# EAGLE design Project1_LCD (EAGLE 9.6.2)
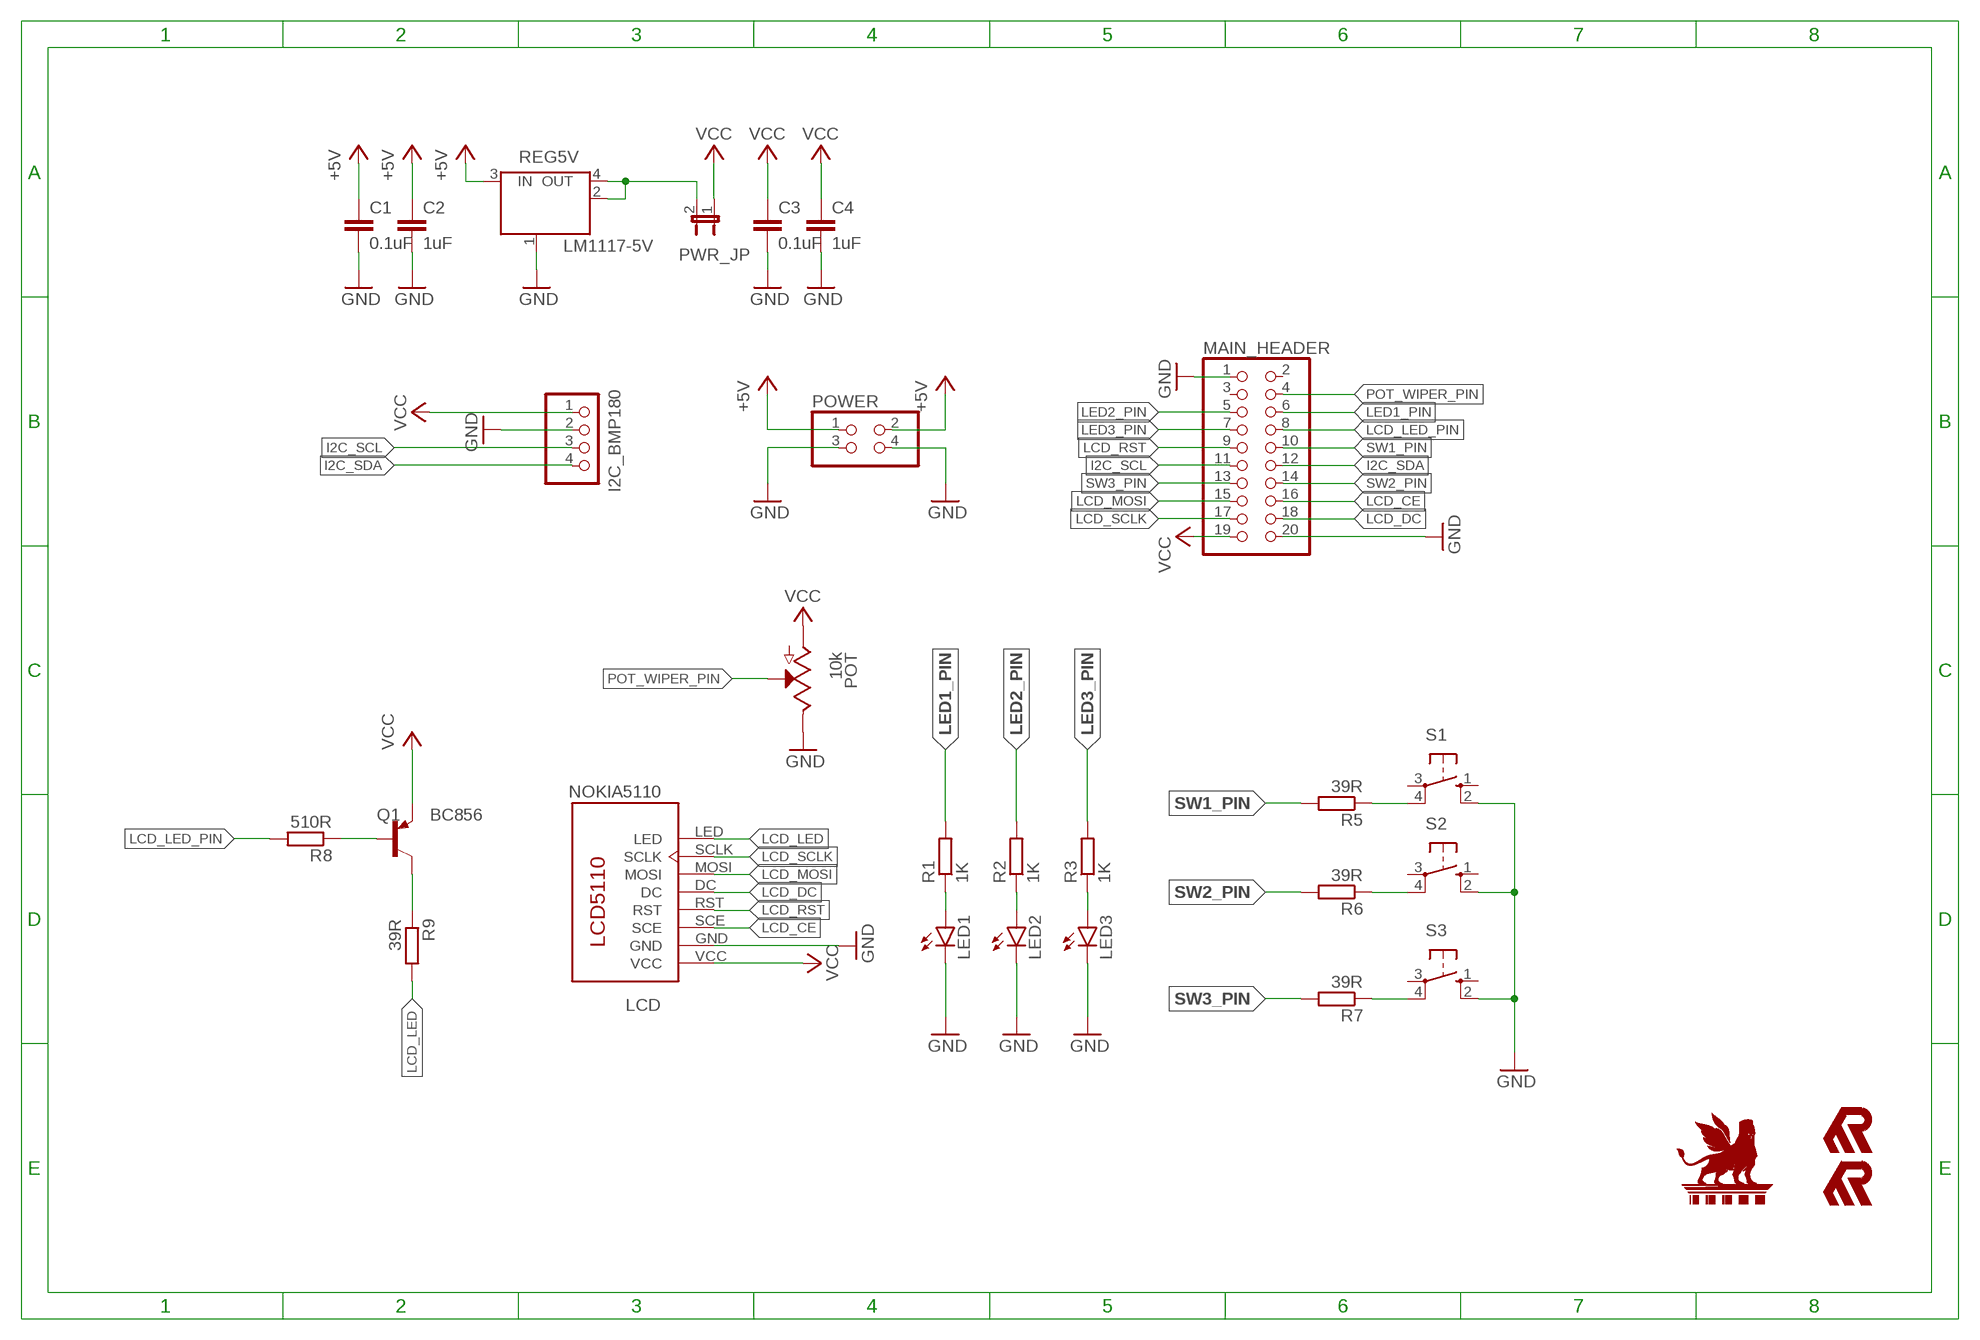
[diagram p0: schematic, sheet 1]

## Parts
C1  0.1uF  C-EUC0805  [C0805]
C2  1uF  C-EUC0805  [C0805]
C3  0.1uF  C-EUC0805  [C0805]
C4  1uF  C-EUC0805  [C0805]
I2C_BMP180  PINHD-1X4  [1X04]
LCD  NOKIA5110  [PCD8544]
LED1  LED5MM  [LED5MM]
LED2  LED5MM  [LED5MM]
LED3  LED5MM  [LED5MM]
MAIN_HEADER  PINHD-2X10  [2X10]
POT  10k  POTENTIOMETER-PTH-9MM-1/20W-20%-KIT  [POT-PTH-ALPS-KIT]
POWER  PINHD-2X2  [2X02]
PWR_JP  JP1E  [JP1]
Q1  BC856  BC856ASMD  [SOT23-BEC]
R1  1K  R-EU_0207/10  [0207/10]
R2  1K  R-EU_0207/10  [0207/10]
R3  1K  R-EU_0207/10  [0207/10]
R5  39R  R-EU_0207/10  [0207/10]
R6  39R  R-EU_0207/10  [0207/10]
R7  39R  R-EU_0207/10  [0207/10]
R8  510R  R-EU_0207/10  [0207/10]
R9  39R  R-EU_0207/10  [0207/10]
REG5V  LM1117-5V  MC33269ST-3.3T3  [SOT223]
S1  40-XX  [B3F-40XX]
S2  40-XX  [B3F-40XX]
S3  40-XX  [B3F-40XX]
U$1  LAMASSU_SMALL_SIZE24  [LAMASSU_SMALL_24MM]
U$2  MR_SMALL_SIZE12  [MR_SMALL_12MM]
U$3  MR_SMALL_SIZE7  [MR_SMALL_7MM]

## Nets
+5V [POWER]: C1.1 C2.1 POWER.1 POWER.2 REG5V.3(IN)
BQ1 [LCD]: Q1.B R8.1
GND [POWER]: C1.2 C2.2 C3.2 C4.2 I2C_BMP180.2 LCD.GND LED1.K(C) LED2.K(C) LED3.K(C) MAIN_HEADER.1 MAIN_HEADER.20 POT.P$1(E) POWER.3 POWER.4 REG5V.1(GND/ADJ) S1.2(S1) S2.2(S1) S3.2(S1)
I2C_SCL: I2C_BMP180.3 MAIN_HEADER.11
I2C_SDA: I2C_BMP180.4 MAIN_HEADER.12
LCD_CE [LCD]: LCD.SCE MAIN_HEADER.16
LCD_DC [LCD]: LCD.DC MAIN_HEADER.18
LCD_LED [LCD]: LCD.LED R9.2
LCD_LED_PIN [LCD]: MAIN_HEADER.8 R8.2
LCD_MOSI [LCD]: LCD.MOSI MAIN_HEADER.15
LCD_RST [LCD]: LCD.RST MAIN_HEADER.9
LCD_SCLK [LCD]: LCD.SCLK MAIN_HEADER.17
LED1_PIN: MAIN_HEADER.6 R1.2
LED2_PIN: MAIN_HEADER.5 R2.2
LED3_PIN: MAIN_HEADER.7 R3.2
N$3: LED3.A R3.1
N$4: LED2.A R2.1
N$5: LED1.A R1.1
N$6: R5.1 S1.4(P1)
N$7: R6.1 S2.4(P1)
N$8: R7.1 S3.4(P1)
POT_WIPER_PIN: MAIN_HEADER.4 POT.P$2(S)
REG_OUT [POWER]: PWR_JP.2 REG5V.2(OUT) REG5V.4(OUT)
RQ1 [LCD]: Q1.C R9.1
SW1_PIN: MAIN_HEADER.10 R5.2
SW2_PIN: MAIN_HEADER.14 R6.2
SW3_PIN: MAIN_HEADER.13 R7.2
VCC [POWER]: C3.1 C4.1 I2C_BMP180.1 LCD.VCC MAIN_HEADER.19 POT.P$3(A) PWR_JP.1 Q1.E
Unconnected: LCD.P$9(NC) LCD.P$10(NC) LCD.P$11(NC) LCD.P$12(NC) LCD.P$13(NC) LCD.P$14(NC) LCD.P$15(NC) LCD.P$16(NC) MAIN_HEADER.2 MAIN_HEADER.3 S1.1(S) S1.3(P) S2.1(S) S2.3(P) S3.1(S) S3.3(P)

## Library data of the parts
C1-C4 = rcl:C-EU: CAPACITOR, European symbol; SPICEPREFIX: C
I2C_BMP180 = pinhead:PINHD-1X4: PIN HEADER
LCD = Rawashdeh_Eagle_Display:NOKIA5110: LCD Nokia 5110 Nokia5110 ased on PCD8544 display driver
LED1-LED3 = led:LED: LED
MAIN_HEADER = pinhead:PINHD-2X10: PIN HEADER
POT = SparkFun-Resistors:POTENTIOMETER: Potentiometer (Pot) Three-terminal potentiometers, with an adjustable wiper and two adjustable resistors. A pot can be used to create a configurable voltage divider, or as a variable resistor. Variants ALPS_POT and ALPS_POT_KIT - PTH, breadboard compatible, 9mm square pots Rotary Potentiometer -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; PROD_ID: RES-09177; SF_SKU: COM-09288
POWER = pinhead:PINHD-2X2: PIN HEADER
PWR_JP = jumper:JP1E: JUMPER
Q1 = transistor-pnp:BC856*: PNP Transistror
R1-R3 R5-R9 = rcl:R-EU_: RESISTOR, European symbol; SPICEPREFIX: R
REG5V = linear:MC33269ST*: Adjustable Output Low Dropout Voltage Regulator 800 mA Source: http://www.onsemi.com/pub/Collateral/MC33269-D.PDF
S1-S3 = switch-omron:40-XX: OMRON SWITCH; MF: OMRON COMPONENTS USA; MPN: B3F-4000; OC_FARNELL: 176434; OC_NEWARK: 36K3105
U$1 = Rawashdeh_Eagle_Logo:LAMASSU_SMALL_SIZE: lamassu Rawashdeh Logo small sizes
U$2 U$3 = Rawashdeh_Eagle_Logo:MR_SMALL_SIZE: MR Mohannad Rawashdeh Logo 7,12 mm

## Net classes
0 default: width 0.254 mm, drill 0.406 mm, clearance 0.305 mm
1 POWER: width 0.406 mm, drill 0.406 mm, clearance 0.305 mm
2 LCD: width 0.254 mm, drill 0.406 mm, clearance 0.305 mm

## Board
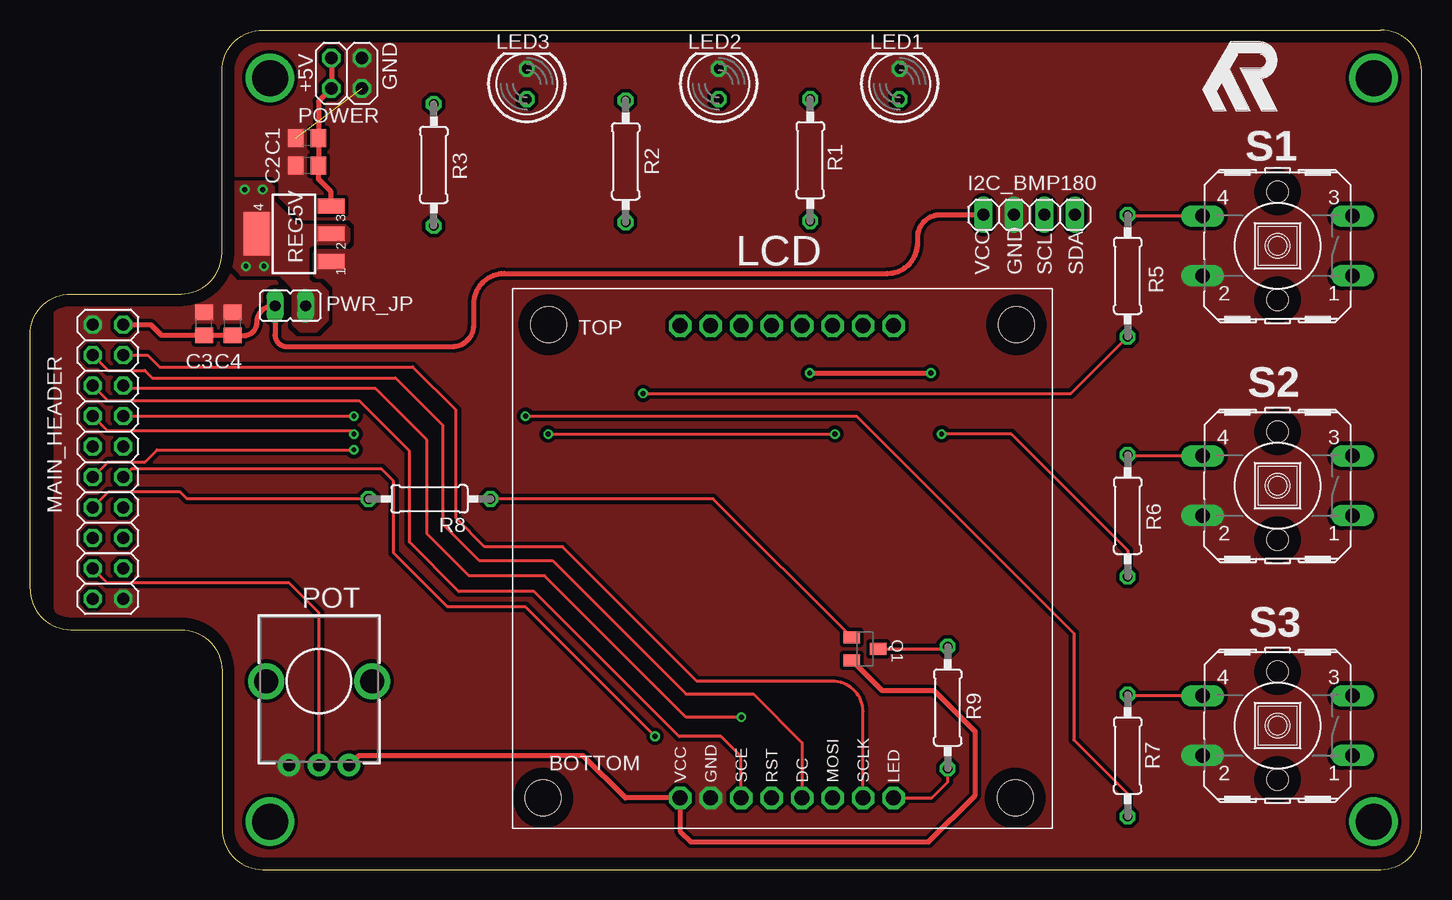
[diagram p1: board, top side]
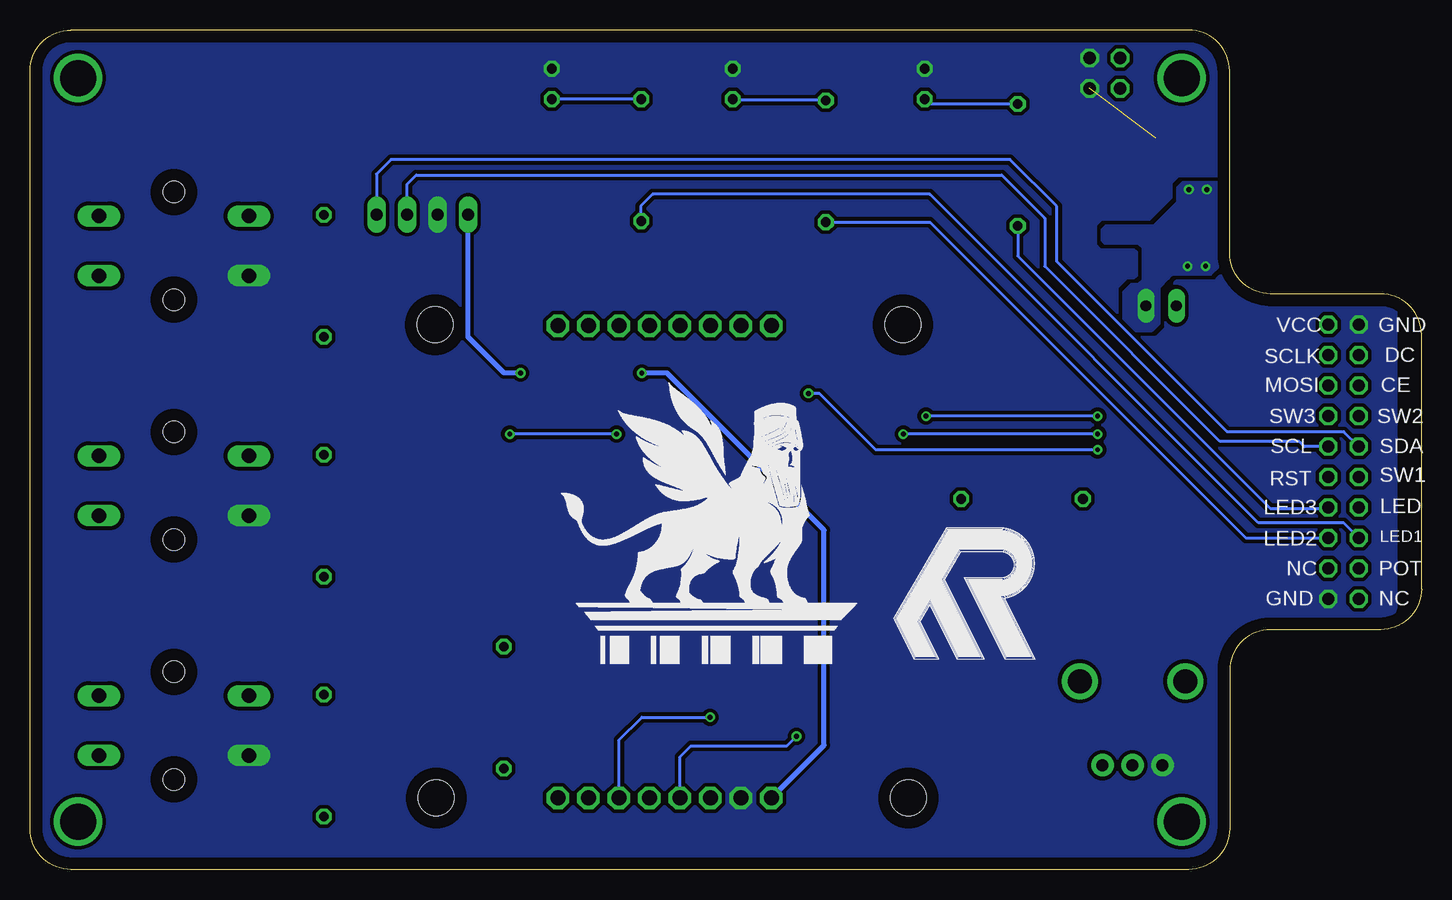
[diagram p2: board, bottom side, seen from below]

Size 116 x 70 mm. Coordinates in mm from the lower left corner, seen from the top.
Outline: 0,23.41 0,44.59 arc-90 3.41,48 12.59,48 arc90 16,51.41 16,66.59 arc-90 19.41,70 112.59,70 arc-90 116,66.59 116,3.41 arc-90 112.59,0 19.41,0 arc-90 16,3.41 16,16.59 arc90 12.59,20 3.41,20 arc-90 0,23.41
Copper layers (1*16): Top 0.035mm / dielectric 1.5mm / Bottom 0.035mm
Design rules "default": minimum track width 6mil, minimum drill 0.35mm, track to track 6mil, track to pad 6mil, pad to pad 6mil, via to via 6mil, smd to smd 6mil, copper to edge 40mil, drill to drill 6mil, minimum pad ring 10mil, minimum via ring 8mil, stop-mask expansion 4mil, vias tented up to drill 0mil, thermal gap 10mil

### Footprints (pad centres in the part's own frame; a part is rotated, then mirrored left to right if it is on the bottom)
C0805 = smd 1.3 x 1.5: 1 -0.95,0; 2 0.95,0
1X04 = drill 1.016 long: 1 -3.81,0; 2 -1.27,0; 3 1.27,0; 4 3.81,0
PCD8544 = drill 1.25 octagon: DC 24.13,2.54; GND 16.51,2.54; LED 31.75,2.54; MOSI 26.67,2.54; P$9 13.97,41.91; P$10 16.51,41.91; P$11 19.05,41.91; P$12 21.59,41.91; P$13 24.13,41.91; P$14 26.67,41.91; P$15 29.21,41.91; P$16 31.75,41.91; RST 21.59,2.54; SCE 19.05,2.54; SCLK 29.21,2.54; VCC 13.97,2.54 | hole 3: 2.54,2.54; 41.91,2.54; 3,42; 42,42
LED5MM = drill 0.813 octagon: A -1.27,0; K 1.27,0
2X10 = drill 1.016 octagon: 1 -11.43,-1.27; 2 -11.43,1.27; 3 -8.89,-1.27; 4 -8.89,1.27; 5 -6.35,-1.27; 6 -6.35,1.27; 7 -3.81,-1.27; 8 -3.81,1.27; 9 -1.27,-1.27; 10 -1.27,1.27; 11 1.27,-1.27; 12 1.27,1.27; 13 3.81,-1.27; 14 3.81,1.27; 15 6.35,-1.27; 16 6.35,1.27; 17 8.89,-1.27; 18 8.89,1.27; 19 11.43,-1.27; 20 11.43,1.27
POT-PTH-ALPS-KIT = drill 1 pad 1.88: P$1 7,-2.5; P$2 7,0; P$3 7,2.5 | drill 2: P$4 0,-4.4; P$5 0,4.4
2X02 = drill 1.016 octagon: 1 -1.27,-1.27; 2 -1.27,1.27; 3 1.27,-1.27; 4 1.27,1.27
JP1 = drill 0.914 long: 1 0,-1.27; 2 0,1.27
SOT23-BEC = smd 1 x 1.4: B -0.95,-1.1; C 0,1.1; E 0.95,-1.1
0207/10 = drill 0.813 octagon: 1 -5.08,0; 2 5.08,0
SOT223 = smd 1.219 x 2.235: 1 -2.311,-3.099; 2 0,-3.099; 3 2.311,-3.099 | smd 3.6 x 2.2: 4 0,3.099
B3F-40XX = drill 1.194 long: 1 -6.248,2.489; 2 6.248,2.489; 3 -6.248,-2.489; 4 6.248,-2.489 | hole 1.803: 0,-4.496; 0,4.496

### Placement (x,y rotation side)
C1  23.1,61 180 top
C2  23.1,58.7 180 top
C3  14.5,45.5 90 top
C4  16.9,45.5 90 top
I2C_BMP180  83.3,54.6 0 top
LCD  40.23,3.43 0 top
LED1  72.5,65.5 90 top
LED2  57.42,65.5 90 top
LED3  41.42,65.5 90 top
MAIN_HEADER  6.5,34 90 top
POT  24.1,15.7 270 top
POWER  26.4,66.4 0 top
PWR_JP  21.7,47 270 top
Q1  69.6,18.4 270 top
R1  65.04,59.15 270 top
R2  49.66,59.05 270 top
R3  33.66,58.75 270 top
R5  91.5,49.5 270 top
R6  91.5,29.5 270 top
R7  91.5,9.5 270 top
R8  33.3,30.9 180 top
R9  76.5,13.5 270 top
REG5V  22,53 90 top
S1  104,52 180 top
S2  104,32 180 top
S3  104,12 180 top
U$1  58.7,23.9 0 bottom
U$2  37,20.9 0 bottom
U$3  101.1,65.9 0 top

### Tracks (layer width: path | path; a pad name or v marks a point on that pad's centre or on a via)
+5V
  Top 0.406: POWER.2 POWER.1 24.05,64.05 C1.1 C2.1 24.05,57.55 25.1,56.5 REG5V.3
BQ1
  Top 0.254: Q1.B 56.95,30.9 R8.1
GND  (1 unrouted)
  pour Top (isolate 0.305, rank 2, no thermals): 3.3,47.7 12.5,47.7 arc90 16.4,51.6 16.4,66.8 arc-90 19.5,69.9 111.9,69.9 arc-90 115.5,66.3 115.5,3.9 arc-90 112,0.4 20.2,0.4 arc-90 16.5,4.1 16.5,16.3 arc90 12.1,20.7 3.5,20.7 arc-90 2.1,22.1 2.1,46.5 arc-90
  pour Bottom (isolate 0.254, rank 2, no thermals): 3.3,47.7 12.5,47.7 arc90 16.4,51.6 16.4,66.8 arc-90 19.5,69.9 111.9,69.9 arc-90 115.5,66.3 115.5,3.9 arc-90 112,0.4 20.2,0.4 arc-90 16.5,4.1 16.5,16.3 arc90 12.1,20.7 3.5,20.7 arc-90 2.1,22.1 2.1,46.5 arc-90
I2C_SCL
  Bottom 0.254: MAIN_HEADER.11 9.77,35.27 10.2,35.7 16.8,35.7 31.4,50.3 31.4,54.3 35,57.9 83.8,57.9 84.57,57.13 I2C_BMP180.3
I2C_SDA
  Bottom 0.254: MAIN_HEADER.12 6.46,36.5 16.2,36.5 30.4,50.7 30.4,55.3 34.3,59.2 85.9,59.2 87.11,57.99 I2C_BMP180.4
LCD_CE
  Top 0.254: MAIN_HEADER.16 6.48,39.1 27.42,39.1 31.63,34.9 31.63,27.3 35.74,23.18 42.04,23.18 54.12,11.1 57.6,11.1 59.28,9.42 LCD.SCE
LCD_DC
  Top 0.254: MAIN_HEADER.18 6.52,41.6 9.56,41.6 10.17,41 30.47,41 34.41,37.06 34.41,28.8 37.45,25.76 43.55,25.76 54.67,14.63 60.31,14.63 64.36,10.58 LCD.DC
LCD_LED
  Top 0.254: LCD.LED 75.17,5.97 76.5,7.3 R9.2
LCD_LED_PIN
  Top 0.254: R8.2 13.1,30.9 12.5,31.5 6.54,31.5 MAIN_HEADER.8
LCD_MOSI  (via drill 0.41)
  Top 0.254: v59.3,12.7 54.7,12.7 42.9,24.5 36.6,24.5 33.1,28 33.1,35.8 28.8,40.1 8.02,40.1 MAIN_HEADER.15
  Bottom 0.254: LCD.MOSI 66.9,10.8 65,12.7 v59.3,12.7
LCD_RST  (via drill 0.41)
  Top 0.254: v52.1,11.1 41.3,21.9 34.8,21.9 30.3,26.4 30.3,32.4 29.3,33.4 8.44,33.4 MAIN_HEADER.9
  Bottom 0.254: LCD.RST 61.82,9.38 60.9,10.3 52.9,10.3 v52.1,11.1
LCD_SCLK
  Top 0.254: LCD.SCLK 69.44,13.16 arc90 66.9,15.7 55.6,15.7 44.4,26.9 37.9,26.9 35.5,29.3 35.5,38.3 31.9,41.9 10.8,41.9 9.81,42.89 MAIN_HEADER.17
LED1_PIN
  Bottom 0.254: MAIN_HEADER.6 6.48,28.9 13.6,28.9 41,56.3 64.1,56.3 65.1,55.3 65.1,54.13 R1.2
LED2_PIN
  Bottom 0.254: R2.2 40.97,53.97 14.65,27.65 MAIN_HEADER.5
LED3_PIN
  Bottom 0.254: R3.2 33.66,51.16 12.6,30.1 7.86,30.1 MAIN_HEADER.7
N$3
  Bottom 0.254: R3.1 41.02,63.83 LED3.A
N$4
  Bottom 0.254: R2.1 57.32,64.13 LED2.A
N$5
  Bottom 0.254: R1.1 LED1.A
N$6
  Top 0.254: S1.4 91.59,54.49 R5.1
N$7
  Top 0.254: S2.4 91.59,34.49 R6.1
N$8
  Top 0.254: S3.4 91.59,14.49 R7.1
N$9  (via drill 3)
  other vias: 112,4
N$10  (via drill 3)
  other vias: 112,66
N$11  (via drill 3)
  other vias: 20,66
N$12  (via drill 3)
  other vias: 20,4
POT_WIPER_PIN
  Top 0.254: POT.P$2 24.1,21.4 21.6,23.9 6.44,23.9 MAIN_HEADER.4
REG_OUT  (via drill 0.41)
  other vias: 18,50.3 19.5,50.3 19.4,56.7 17.9,56.7
  pour Top (isolate 0.406, no thermals): 26.1,53.7 23.6,53.7 22.3,53.7 20.9,55.1 20.3,55.7 20.3,56.1 20.3,56.9 20.1,57.1 19.9,57.3 16.7,57.3 16.6,57.3 16.3,57 16.3,50.9 17,50.2 17.6,49.6 19.5,49.6 20.8,49.6 21.1,49.3 21.9,48.5 21.9,47.8 21.9,45.5 22.5,44.9 23.4,44.9 23.9,44.9 24.8,45.8 24.8,48.2 24.2,48.8 23.6,48.8 23.2,49.2 23.2,50.8 23.2,51.8 23.6,52.2 26.4,52.2 26.5,52.3 26.6,52.4 26.6,53.4 26.3,53.7
  pour Bottom (isolate 0.254, no thermals): 26.1,53.7 23.6,53.7 22.3,53.7 20.9,55.1 20.3,55.7 20.3,56.1 20.3,56.9 20.1,57.1 19.9,57.3 16.7,57.3 16.6,57.3 16.3,57 16.3,50.9 17,50.2 17.6,49.6 19.5,49.6 20.8,49.6 21.1,49.3 21.9,48.5 21.9,47.8 21.9,45.5 22.5,44.9 23.4,44.9 23.9,44.9 24.8,45.8 24.8,48.2 24.2,48.8 23.6,48.8 23.2,49.2 23.2,50.8 23.2,51.8 23.6,52.2 26.4,52.2 26.5,52.3 26.6,52.4 26.6,53.4 26.3,53.7
RQ1
  Top 0.254: Q1.C 76.32,18.4 R9.1
SW1_PIN  (via drill 0.41)
  Top 0.254: MAIN_HEADER.10 6.5,34 9.6,34 10.6,35 v27,35 | v51.1,39.7 86.78,39.7 R5.2
  Bottom 0.254: v27,35 45.5,35 50.2,39.7 v51.1,39.7
SW2_PIN  (via drill 0.41)
  Top 0.254: MAIN_HEADER.14 6.44,36.6 26.7,36.6 v27,36.3 | v76,36.3 81.8,36.3 91.5,26.6 R6.2 | v43.2,36.3 v67.1,36.3
  Bottom 0.254: v27,36.3 v43.2,36.3 | v67.1,36.3 v76,36.3
SW3_PIN  (via drill 0.41)
  Top 0.254: MAIN_HEADER.13 v26.99,37.81 v27,37.8 | v41.3,37.8 68.9,37.8 87,19.7 87,10.8 91.5,6.3 R7.2
  Bottom 0.254: v27,37.8 v41.3,37.8
VCC  (via drill 0.41)
  Top 0.406: MAIN_HEADER.19 10.07,45.43 10.95,44.55 C3.1 C4.1 arc90 16.95,44.5 17.8,44.5 arc90 18.9,45.6 arc-90 20.3,47 PWR_JP.1 20.43,44.57 arc90 21.4,43.6 35.2,43.6 arc90 37,45.4 37,47.16 arc-90 39.54,49.7 71.46,49.7 arc90 74,52.24 74,52.7 arc-90 75.9,54.6 I2C_BMP180.1 | POT.P$3 27.4,9.5 46.1,9.5 49.63,5.97 LCD.VCC 54.2,3.2 55.1,2.3 74.9,2.3 78.8,6.2 78.8,11.5 75.4,14.9 71.05,14.9 Q1.E | v65,41.4 v75.1,41.4
  Bottom 0.406: LCD.VCC 49.8,10.37 49.8,28.3 62.9,41.4 v65,41.4 | I2C_BMP180.1 79.5,44.4 76.5,41.4 v75.1,41.4

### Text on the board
tNames: +5V | GND | VCC | GND | SCL | SDA
bNames: GND | VCC | DC | SCLK | CE | MOSI | SW2 | SW3 | SDA | SCL | SW1 | RST | LED | LED3 | LED1 | LED2 | POT | NC | NC | GND

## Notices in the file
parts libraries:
SparkFun-Resistors: Licensing: Creative Commons ShareAlike 4.0 International - https://creativecommons.org/licenses/by-sa/4.0
